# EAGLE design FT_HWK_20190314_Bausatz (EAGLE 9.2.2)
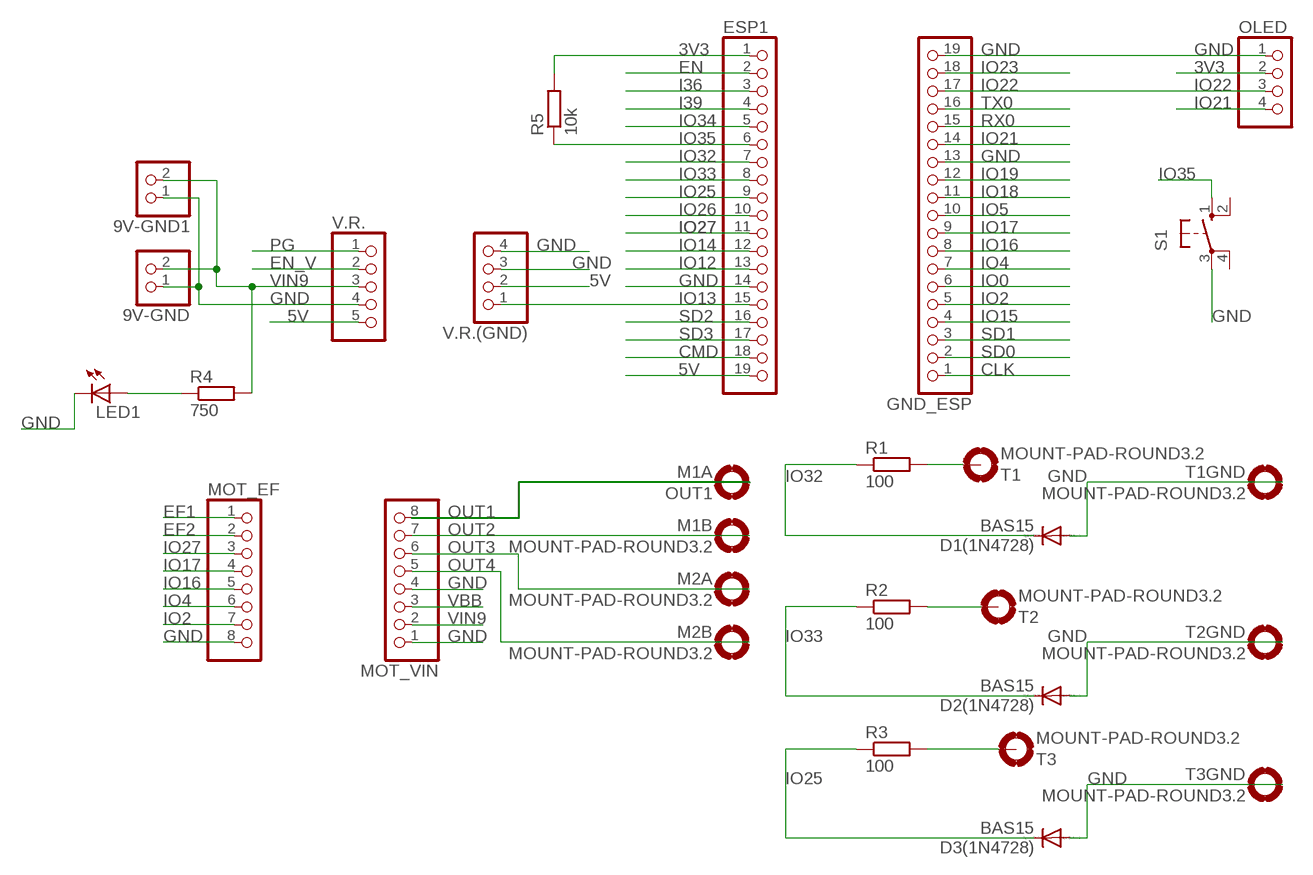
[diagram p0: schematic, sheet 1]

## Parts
9V-GND  PINHD-1X2  [1X02]
9V-GND1  PINHD-1X2  [1X02]
D1(1N4728)  BAS15  [DO34-7]
D2(1N4728)  BAS15  [DO34-7]
D3(1N4728)  BAS15  [DO34-7]
ESP1  PINHD-1X19  [1X19]
GND_ESP  PINHD-1X19  [1X19]
LED1  LED3MM  [LED3MM]
M1A  OUT1  MOUNT-PAD-ROUND3.2  [3,2-PAD]
M1B  MOUNT-PAD-ROUND3.2  [3,2-PAD]
M2A  MOUNT-PAD-ROUND3.2  [3,2-PAD]
M2B  MOUNT-PAD-ROUND3.2  [3,2-PAD]
MOT_EF  PINHD-1X8  [1X08]
MOT_VIN  PINHD-1X8  [1X08]
OLED  PINHD-1X4  [1X04]
R1  100  R-EU_0207/5V  [0207/5V]
R2  100  R-EU_0207/5V  [0207/5V]
R3  100  R-EU_0207/5V  [0207/5V]
R4  750  R-EU_0207/5V  [0207/5V]
R5  10k  R-EU_0207/5V  [0207/5V]
S1  10-XX  [B3F-10XX]
T1  MOUNT-PAD-ROUND3.2  [3,2-PAD]
T1GND  MOUNT-PAD-ROUND3.2  [3,2-PAD]
T2  MOUNT-PAD-ROUND3.2  [3,2-PAD]
T2GND  MOUNT-PAD-ROUND3.2  [3,2-PAD]
T3  MOUNT-PAD-ROUND3.2  [3,2-PAD]
T3GND  MOUNT-PAD-ROUND3.2  [3,2-PAD]
V.R.  PINHD-1X5  [1X05]
V.R.(GND)  PINHD-1X4  [1X04]

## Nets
3V3: ESP1.1 OLED.2 R5.2
5V: ESP1.19 V.R.(GND).2 V.R..5
CLK: GND_ESP.1
CMD: ESP1.18
EF1: MOT_EF.1
EF2: MOT_EF.2
EN: ESP1.2
EN_V: V.R..2
GND [MOT_OUT]: 9V-GND1.1 9V-GND.1 D1(1N4728).A D2(1N4728).A D3(1N4728).A ESP1.14 GND_ESP.13 GND_ESP.19 LED1.K(C) MOT_EF.8 MOT_VIN.1 MOT_VIN.4 OLED.1 S1.3(P) T1GND.BH3,2(MOUNT) T2GND.BH3,2(MOUNT) T3GND.BH3,2(MOUNT) V.R.(GND).3 V.R.(GND).4 V.R..4
I36: ESP1.3
I39: ESP1.4
IO0: GND_ESP.6
IO2: GND_ESP.5 MOT_EF.7
IO4: GND_ESP.7 MOT_EF.6
IO5: GND_ESP.10
IO12: ESP1.13
IO13: ESP1.15 V.R.(GND).1
IO14: ESP1.12
IO15: GND_ESP.4
IO16: GND_ESP.8 MOT_EF.5
IO17: GND_ESP.9 MOT_EF.4
IO18: GND_ESP.11
IO19: GND_ESP.12
IO21: GND_ESP.14 OLED.4
IO22: GND_ESP.17 OLED.3
IO23: GND_ESP.18
IO25: D3(1N4728).C ESP1.9 R3.1
IO26: ESP1.10
IO27: ESP1.11 MOT_EF.3
IO32: D1(1N4728).C ESP1.7 R1.1
IO33: D2(1N4728).C ESP1.8 R2.1
IO34: ESP1.5
IO35: ESP1.6 R5.1 S1.1(S)
N$1: LED1.A R4.1
N$2: R1.2 T1.BH3,2(MOUNT)
N$3: R2.2 T2.BH3,2(MOUNT)
N$4: R3.2 T3.BH3,2(MOUNT)
OUT1 [MOT_OUT]: M1A.BH3,2(MOUNT) MOT_VIN.8
OUT2 [MOT_OUT]: M1B.BH3,2(MOUNT) MOT_VIN.7
OUT3 [MOT_OUT]: M2A.BH3,2(MOUNT) MOT_VIN.6
OUT4 [MOT_OUT]: M2B.BH3,2(MOUNT) MOT_VIN.5
PG: V.R..1
RX0: GND_ESP.15
SD0: GND_ESP.2
SD1: GND_ESP.3
SD2: ESP1.16
SD3: ESP1.17
TX0: GND_ESP.16
VBB: MOT_VIN.3
VIN9 [MOT_OUT]: 9V-GND1.2 9V-GND.2 MOT_VIN.2 R4.2 V.R..3
Unconnected: S1.2(S1) S1.4(P1)

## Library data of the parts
9V-GND 9V-GND1 = pinhead:PINHD-1X2: PIN HEADER
D1(1N4728) D2(1N4728) D3(1N4728) = diode:BAS15: DIODE
ESP1 = pinhead:PINHD-1X19: PIN HEADER
GND_ESP = pinhead:PINHD-1X19: PIN HEADER; SPICEPREFIX: X
LED1 = led:LED: LED
M1A M1B M2A M2B T1 T1GND T2 T2GND T3 T3GND = Walter:MOUNT-PAD-ROUND: MOUNTING PAD, round
MOT_EF MOT_VIN = pinhead:PINHD-1X8: PIN HEADER
OLED V.R.(GND) = pinhead:PINHD-1X4: PIN HEADER
R1-R5 = rcl:R-EU_: RESISTOR, European symbol; SPICEPREFIX: R
S1 = switch-omron:10-XX: OMRON SWITCH; MPN: B3F-1000; OC_FARNELL: 176432; OC_NEWARK: 36M3542
V.R. = pinhead:PINHD-1X5: PIN HEADER

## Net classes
0 default: clearance 0.305 mm
1 MOT_OUT: width 0.6 mm, clearance 0.305 mm to class 0, clearance 0.305 mm

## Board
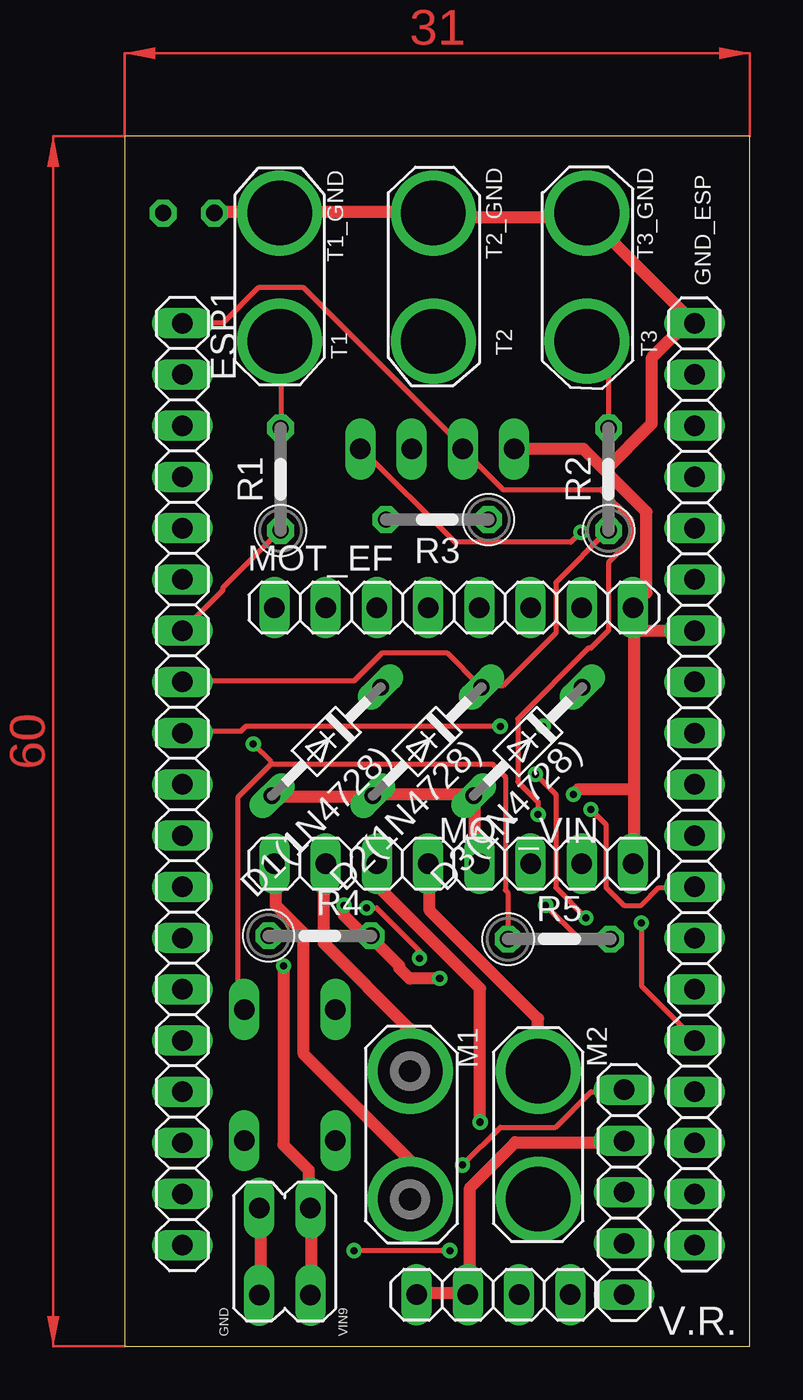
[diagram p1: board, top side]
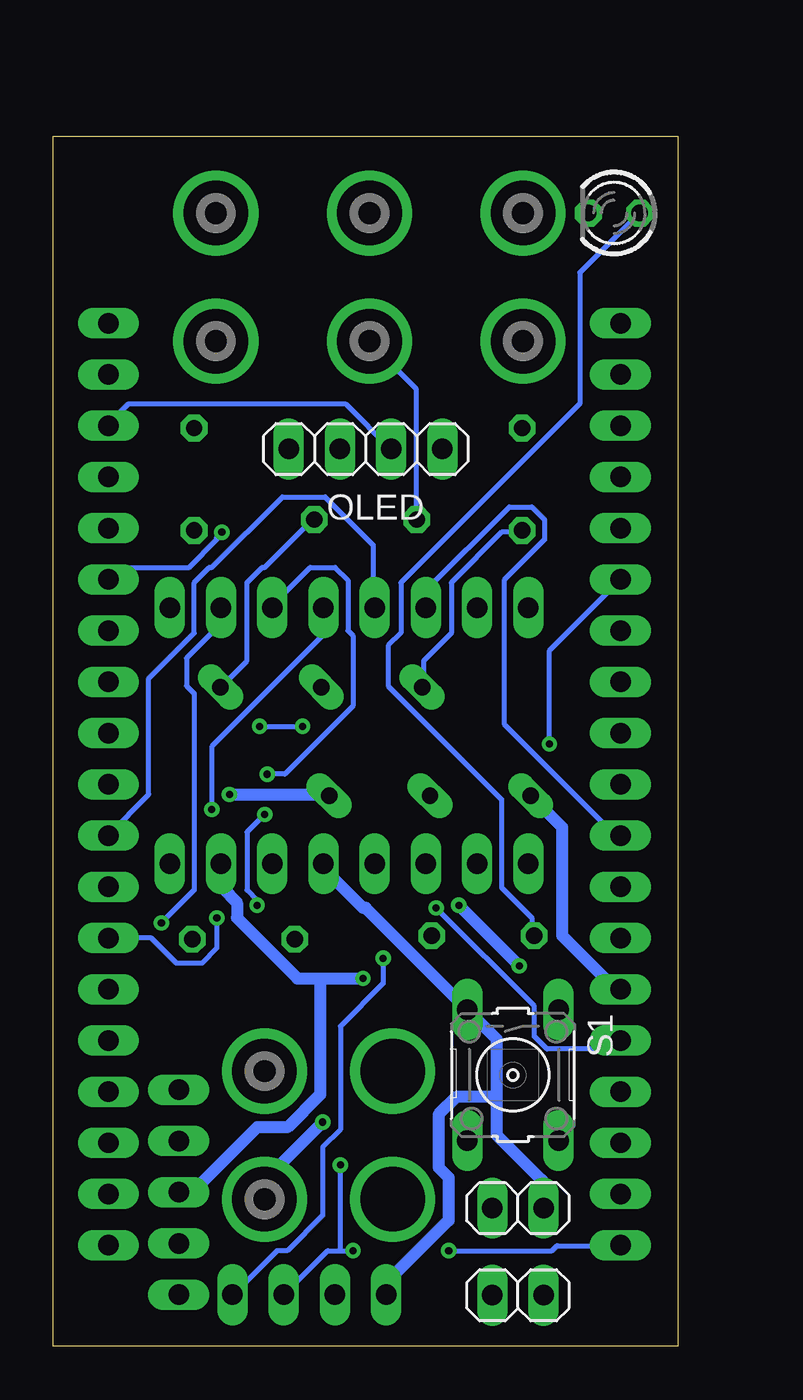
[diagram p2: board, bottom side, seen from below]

Size 31 x 60 mm. Coordinates in mm from the lower left corner, seen from the top.
Outline: 0,0 31,0 31,60 0,60 0,0
Copper layers (1*16): Top 0.035mm / dielectric 1.5mm / Bottom 0.035mm
Design rules "default *": minimum track width 10mil, minimum drill 0.35mm, track to track 6mil, track to pad 6mil, pad to pad 6mil, via to via 6mil, smd to smd 6mil, copper to edge 40mil, drill to drill 6mil, minimum pad ring 10mil, minimum via ring 8mil, stop-mask expansion 4mil, vias tented up to drill 0mil, thermal gap 10mil

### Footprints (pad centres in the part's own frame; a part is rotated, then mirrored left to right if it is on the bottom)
1X02 = drill 1.016 long: 1 -1.27,0; 2 1.27,0
DO34-7 = drill 0.813 long: A 3.81,0; C -3.81,0
1X19 = drill 1.016 long: 1 -22.86,0; 2 -20.32,0; 3 -17.78,0; 4 -15.24,0; 5 -12.7,0; 6 -10.16,0; 7 -7.62,0; 8 -5.08,0; 9 -2.54,0; 10 0,0; 11 2.54,0; 12 5.08,0; 13 7.62,0; 14 10.16,0; 15 12.7,0; 16 15.24,0; 17 17.78,0; 18 20.32,0; 19 22.86,0
LED3MM = drill 0.813 octagon: A -1.27,0; K 1.27,0
3,2-PAD = drill 3.2 pad 3.81: BH3,2 0,0
1X08 = drill 1.016 long: 1 -8.89,0; 2 -6.35,0; 3 -3.81,0; 4 -1.27,0; 5 1.27,0; 6 3.81,0; 7 6.35,0; 8 8.89,0
1X04 = drill 1.016 long: 1 -3.81,0; 2 -1.27,0; 3 1.27,0; 4 3.81,0
0207/5V = drill 0.813 octagon: 1 -2.54,0; 2 2.54,0
B3F-10XX = drill 1.016 long: 1 -3.251,2.261; 2 3.251,2.261; 3 -3.251,-2.261; 4 3.251,-2.261
1X05 = drill 1.016 long: 1 -5.08,0; 2 -2.54,0; 3 0,0; 4 2.54,0; 5 5.08,0

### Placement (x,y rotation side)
9V-GND  7.94,2.54 180 bottom
9V-GND1  7.94,6.86 180 bottom
D1(1N4728)  10,30 225 top
D2(1N4728)  15,30 225 top
D3(1N4728)  20,30 225 top
ESP1  2.86,27.88 270 top
GND_ESP  28.26,27.88 90 top
LED1  3.17,56.2 180 bottom
M1A  14.16,7.3 180 top
M1B  14.16,13.65 180 top
M2A  20.51,7.3 0 bottom
M2B  20.51,13.65 0 bottom
MOT_EF  16.32,36.64 0 top
MOT_VIN  16.32,23.94 180 top
OLED  15.5,44.5 0 bottom
R1  7.73,43 90 top
R2  24,43 90 top
R3  15.5,41 180 top
R4  9.68,20.37 0 top
R5  21.55,20.2 0 top
S1  8.19,13.46 270 bottom
T1  7.68,49.85 0 bottom
T1GND  7.68,56.2 180 bottom
T2  22.92,49.85 0 bottom
T2GND  22.92,56.2 0 bottom
T3  15.3,49.85 0 bottom
T3GND  15.3,56.2 0 bottom
V.R.  24.77,7.65 90 top
V.R.(GND)  18.29,2.57 180 top

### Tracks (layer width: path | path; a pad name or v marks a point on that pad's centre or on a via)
3V3  (via drill 0.35)
  Top 0.254: v20.88,21.88 22.5,20.25 24,20.25 R5.2 | v20.5,26.38 20.5,27 19.5,28 19.5,31.12 23,34.62 23.12,34.62 24,35.5 24,38.88 25.12,40 25.12,41 23.62,42.5 18.75,42.5 16.75,44.5 OLED.2 16.75,44.62 8.88,52.5 6.62,52.5 4.88,50.75 2.88,50.75 ESP1.1
  Bottom 0.254: v20.88,21.88 20.88,22.12 21.38,22.62 21.38,25.5 v20.5,26.38
5V  (via drill 0.35)
  Top 0.254: v16.12,4.75 v11.38,4.75 | v16.75,9 18.62,10.88 21.38,10.88 23.12,12.62 24.75,12.62 V.R..5
  Bottom 0.254: v11.38,4.75 6.25,4.75 6,5 2.88,5 ESP1.19 | 16.75,4.75 17.38,4.75 19.5,2.62 V.R.(GND).2 | 16.75,4.75 v16.12,4.75 | 16.75,4.75 v16.75,9
GND  (via drill 0.35)
  Top 0.6: D1(1N4728).A 7.38,27.25 12.25,27.25 D2(1N4728).A 12.5,27.38 17,27.38 D3(1N4728).A 17.38,27.25 17.38,24.12 17.5,24 MOT_VIN.4 | V.R.(GND).4 14.5,2.62 17,2.62 V.R.(GND).3 17.12,2.88 17.12,7.88 19.38,10.12 24.75,10.12 V.R..4 | 9V-GND.1 6.75,2.62 6.75,6.75 9V-GND1.1 | 25.25,27.62 25.25,36.62 MOT_EF.8 | 25.25,27.62 25.25,24 MOT_VIN.1 | OLED.1 22.75,44.5 23.81,43.44 | 23.81,43.44 25.88,41.38 25.88,37.38 25.38,36.88 MOT_EF.8 | GND_ESP.13 25.5,35.5 MOT_EF.8 | LED1.K 4.5,56.25 7.62,56.25 T1GND.BH3,2 7.88,56.25 15.25,56.25 T3GND.BH3,2 15.5,56 22.62,56 T2GND.BH3,2 22.88,56.12 GND_ESP.19 27.88,50.75 26.12,49 26.12,45.75 23.81,43.44 | v22.25,27.38 22.5,27.62 25.25,27.62
  Bottom 0.6: D1(1N4728).A 5.75,25.75 5.75,20.38 3.12,17.75 2.88,17.75 ESP1.14 | MOT_VIN.4 17.5,23.88 17.5,23.62 15.62,21.75 15.5,21.75 10.5,16.75 S1.3 10.25,16.5 9,15.25 9,12.38 | 9,12.38 9,10.5 6.75,8.25 6.75,6.88 9V-GND1.1 | 9,12.38 11,12.38 11.88,11.5 11.88,8.88 11.38,8.38 11.38,6.25 14.38,3.25 14.38,2.62 V.R.(GND).4 | v22.25,27.38 17.38,27.38 D3(1N4728).A
IO2  (via drill 0.35)
  Top 0.254: v25.62,21 25.62,17.88 28.25,15.25 GND_ESP.5
  Bottom 0.254: v25.62,21 24,22.62 24,32.38 24.38,32.75 24.38,34.12 22.75,35.75 22.75,36.62 MOT_EF.7
IO4  (via drill 0.35)
  Top 0.254: v22.88,21.25 21.38,22.75 21.38,27.38 v20.38,28.38
  Bottom 0.254: v22.88,21.25 22.88,19.75 23.62,19 24.88,19 26.12,20.25 GND_ESP.7 | v20.38,28.38 19.5,28.38 16.12,31.75 16.12,35.25 16.38,35.5 16.38,38 17,38.62 18.25,38.62 20.12,36.75 MOT_EF.6
IO13  (via drill 0.35)
  Top 0.254: v14.62,19.25 14.62,19.62 12.5,21.75 v12,21.75
  Bottom 0.254: v14.62,19.25 14.62,18 16.75,15.88 16.75,10.75 17.62,9.88 17.62,6.5 19.38,4.75 19.88,4.75 22,2.62 V.R.(GND).1 | v12,21.75 7.12,16.88 7.12,15.38 6.5,14.75 3.25,14.75 2.88,15.12 ESP1.15
IO16  (via drill 0.35)
  Top 0.254: v23.12,26.62 23.88,25.88 23.88,22.75 24.75,21.88 25.62,21.88 26.5,22.75 28.25,22.75 GND_ESP.8
  Bottom 0.254: v23.12,26.62 23.12,29.75 17.62,35.25 17.62,36.62 MOT_EF.5
IO17
  Bottom 0.254: MOT_EF.4 15.12,36.75 15.12,39.75 17.5,42.12 19.62,42.12 23.12,38.62 23.25,38.62 24,37.88 24,35.38 26.25,33.12 26.25,27.38 28.25,25.38 GND_ESP.9
IO21  (via drill 0.35)
  Top 0.254: v22.62,40.38 22.12,39.88 16.38,39.88 11.75,44.5 OLED.4
  Bottom 0.254: v22.62,40.38 22.88,40.12 22.88,40 24.25,38.62 27.75,38.62 28.25,38.12 GND_ESP.14
IO22
  Bottom 0.254: OLED.3 14.25,44.5 16.5,46.75 27.25,46.75 28.25,45.75 GND_ESP.17
IO25  (via drill 0.35)
  Top 0.254: v18.62,30.75 6,30.75 5.75,30.5 2.88,30.5 ESP1.9 | D3(1N4728).C v20.75,30.75
  Bottom 0.254: R3.1 18.12,41 20.5,38.62 20.62,38.62 21.38,37.88 21.38,34 22.62,32.75 D3(1N4728).C | v20.75,30.75 v18.62,30.75
IO27
  Bottom 0.254: ESP1.11 2.88,25.38 3.12,25.38 8.62,30.88 8.62,38 6.62,40 6.62,41 7.25,41.62 8.38,41.62 12.5,37.5 12.5,36.75 MOT_EF.3
IO32
  Top 0.254: R1.1 7.62,40.38 4.88,37.62 4.88,37.5 2.88,35.5 ESP1.7
  Bottom 0.254: D1(1N4728).C 12.62,32.75 12.62,34 11.25,35.38 11.25,37.88 8.75,40.38 7.75,40.38 R1.1
IO33
  Top 0.254: R2.1 24,40.5 21.38,37.88 21.38,35.38 18.75,32.75 17.75,32.75 D2(1N4728).C 17.62,32.75 16,34.38 12.75,34.38 11.38,33 2.88,33 ESP1.8
IO35  (via drill 0.35)
  Top 0.254: 7.25,28.88 18.25,28.88 18.88,28.25 18.88,22.62 19,22.5 19,20.25 R5.1 | 7.25,28.88 5.62,27.25 5.62,17 5.88,16.75 S1.1 | v6.38,29.88 7.25,29 7.25,28.88
  Bottom 0.254: v6.38,29.88 6.38,34.5 2.88,38 ESP1.6
N$1
  Bottom 0.254: R4.1 7.25,20.38 7.25,21.25 8.75,22.75 8.75,27.12 14.38,32.75 14.38,34.75 13.75,35.38 13.75,37.88 4.88,46.75 4.88,53.25 2,56.12 LED1.A
N$2
  Top 0.254: R1.2 7.75,45.62 7.75,49.75 T1.BH3,2
N$3
  Top 0.254: R2.2 24,48.75 23,49.75 T2.BH3,2
N$4
  Bottom 0.254: R3.2 13,41 13,47.5 15.25,49.75 T3.BH3,2
OUT1
  Top 0.6: MOT_VIN.8 7.5,23.88 7.5,21.88 8.88,20.5 8.88,14.5 14.12,9.25 14.12,7.38 M1A.BH3,2
OUT2
  Top 0.6: MOT_VIN.7 9.88,23.88 9.88,20 14.12,15.75 14.12,13.75 M1B.BH3,2
OUT3  (via drill 0.35)
  Top 0.6: v17.62,11.12 17.62,17.75 12.62,22.75 12.62,23.88 MOT_VIN.6
  Bottom 0.6: v17.62,11.12 20.5,8.25 20.5,7.38 M2A.BH3,2
OUT4
  Top 0.6: MOT_VIN.5 15.12,23.88 15.12,21.62 20.5,16.25 20.5,13.75 M2B.BH3,2
VIN9  (via drill 0.35)
  Top 0.6: 9V-GND.2 9.25,2.62 9.25,6.75 9V-GND1.2 9.12,7.12 9.12,8.75 7.88,10 v7.88,18.88 | v15.62,18.25 14.12,18.25 13.62,18.75 13.62,18.88 12.25,20.25 R4.2 12,20.25 10.88,21.38 v10.88,21.88
  Bottom 0.6: 17.75,18.25 18.88,18.25 21.88,21.25 21.88,22 22.62,22.75 22.62,23.88 MOT_VIN.2 | 17.75,18.25 v15.62,18.25 | 17.75,18.25 17.75,12.5 19.38,10.88 20.88,10.88 24,7.75 24.75,7.75 V.R..3 | v10.88,21.88 v7.88,18.88
(copper drawn outside any net)
  shapes: Top area x2

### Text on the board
tNames: T1_GND | T2_GND | T3_GND | T2 | T1 | T3 | M1 | M2 | GND | VIN9 | V.R.
Beschriftung_Bottom: M1 | M2 | T1 | T2 | T3 | GND | 9V | FT-Mini-ESP32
